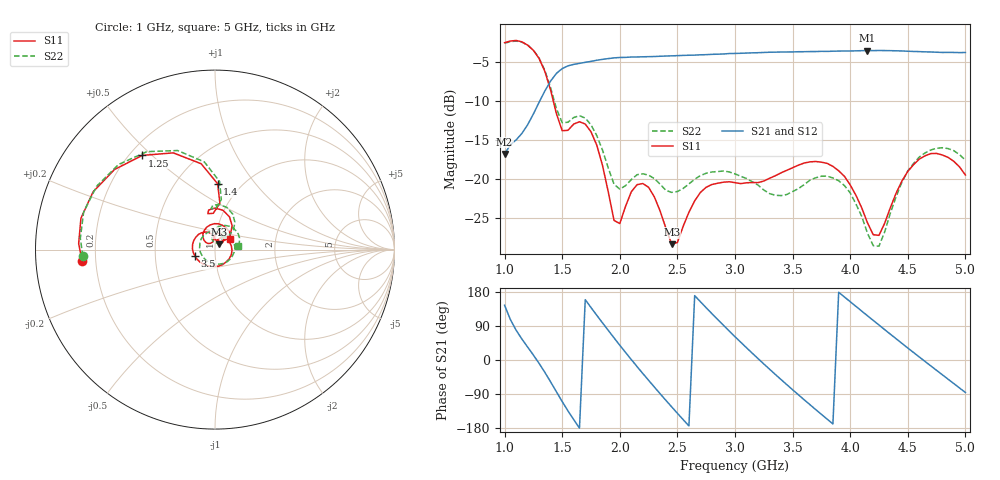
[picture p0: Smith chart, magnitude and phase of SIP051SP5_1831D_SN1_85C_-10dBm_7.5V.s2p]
# GHz  S  dB  R  50
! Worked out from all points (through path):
!   81 points, 1 GHz to 5 GHz, reference 50 ohm
!   highest |S21| = -3.59 dB at 4.15 GHz (marker M1); lowest = -16.8 dB at 1 GHz (marker M2)
!   lowest |S11| = -28.4 dB at 2.45 GHz (marker M3), VSWR 1.08, Z = 52.3 + j3.15 ohm
!   |S11| at or under -10 dB: 1.422 GHz to end of sweep
!   |S22| runs from -28.7 to -2.4 dB; largest |S21 - S12| = 0.0018
!   S11 on the Smith chart (normalised r, x): 1 GHz: 0.15, -0.04; 1.25 GHz: 0.25, +0.47; 1.4 GHz: 0.78, +0.66; 3.5 GHz: 0.80, -0.06; 5 GHz: 1.18, +0.15
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1  -2.59 -174.9  -16.84 144.3  -16.84 144.4  -2.65 -177.2
1.25  -3.57 127.7  -11.72 13.0  -11.71 12.8  -3.55 124.8
1.4  -8.70 87.7  -7.48 -58.0  -7.46 -58.0  -8.39 86.2
1.5  -13.87 92.7  -5.91 -109.8  -5.89 -109.7  -12.84 89.4
1.7  -13.01 78.4  -5.11 159.2  -5.10 159.2  -12.24 74.2
1.85  -18.32 44.9  -4.72 97.9  -4.71 97.9  -16.35 47.2
1.95  -25.36 54.8  -4.54 58.4  -4.54 58.3  -20.73 51.1
2.05  -23.55 92.9  -4.47 19.9  -4.46 20.0  -20.90 69.2
2.2  -20.64 69.8  -4.40 -35.7  -4.39 -35.7  -19.39 60.9
2.35  -24.16 43.6  -4.33 -89.0  -4.32 -89.0  -20.72 48.4
2.45  -28.39 52.2  -4.28 -123.6  -4.26 -123.6  -21.77 49.4
2.7  -21.77 53.8  -4.14 153.7  -4.13 153.8  -19.61 41.2
2.85  -20.60 12.3  -4.06 106.7  -4.05 106.7  -19.09 19.0
3  -20.52 -32.9  -3.97 61.5  -3.95 61.5  -19.39 -8.7
3.25  -20.31 -105.1  -3.84 -10.4  -3.84 -10.3  -21.47 -73.3
3.5  -18.61 -161.2  -3.78 -78.4  -3.77 -78.5  -21.66 -168.2
3.7  -17.81 157.5  -3.73 -130.6  -3.72 -130.7  -19.90 128.1
3.9  -19.00 119.3  -3.67 178.8  -3.66 178.8  -20.27 80.4
4.15  -25.66 98.3  -3.59 116.8  -3.59 116.7  -27.00 54.2
4.35  -23.67 141.8  -3.61 67.8  -3.61 67.8  -24.36 106.4
4.65  -17.08 100.8  -3.76 -3.8  -3.76 -4.0  -16.71 67.2
5  -19.55 35.9  -3.85 -85.7  -3.85 -85.8  -17.62 9.4
